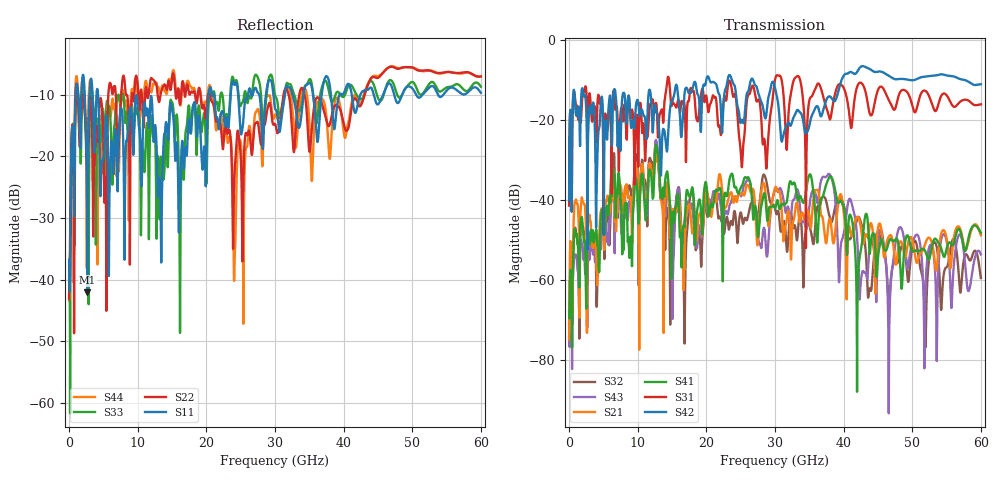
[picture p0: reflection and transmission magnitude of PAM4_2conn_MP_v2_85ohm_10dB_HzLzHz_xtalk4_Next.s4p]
! Info: Touchstone file created by Circ.  Input file=FAB50GbE_2conn_Midplane_Examax_Topo2_v2_85ohm_10dB_HzLzHz.circ
# Hz S RI R 50
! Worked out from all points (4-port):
!   6000 points, 10 MHz to 60 GHz, reference 50 ohm
!   strongest paths, dB at 10 MHz, 15.01 GHz, 30.01 GHz, 45.01 GHz, 60 GHz:
!     S42: -40.1, -15.4, -12.0, -8.0, -11.2
!     S31: -41.4, -16.0, -10.0, -12.6, -16.1
!     S41: -67.8, -45.3, -42.0, -54.4, -48.1
!     S21: -74.8, -45.4, -37.0, -47.0, -48.8
!     S43: -70.7, -59.4, -37.3, -51.7, -53.6
!     S32: -74.2, -59.0, -42.0, -48.0, -59.4
!   lowest |S11| = -42.0 dB at 2.68 GHz (marker M1), VSWR 1.02, Z = 49.3 + j0.404 ohm
!   |S11| at or under -10 dB: 4.23 GHz to 20.31 GHz (16.08 GHz wide, 131 % of centre); 21.13 GHz to 23.54 GHz (2.41 GHz wide, 10.8 % of centre); 29.77 GHz to 31.44 GHz (1.67 GHz wide, 5.46 % of centre)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
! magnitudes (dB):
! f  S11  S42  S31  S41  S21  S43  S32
! 10 MHz  -40.1  -40.1  -41.4  -67.8  -74.8  -70.7  -74.2
! 1.19 GHz  -8.4  -18.7  -17.3  -49.8  -40.9  -56.5  -50.3
! 2.68 GHz  -42.0  -52.5  -21.8  -48.1  -49.7  -59.9  -63.2
! 12.73 GHz  -17.8  -18.0  -16.2  -26.5  -28.2  -25.3  -25.9
! 16.78 GHz  -21.2  -14.3  -15.8  -46.8  -56.6  -45.7  -68.9
! 28.42 GHz  -14.0  -18.6  -24.7  -38.3  -35.9  -47.0  -33.7
! 60 GHz  -9.7  -11.2  -16.1  -48.1  -48.8  -53.6  -59.4
